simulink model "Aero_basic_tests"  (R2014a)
settings: Solver=ode1  StartTime=0.0  StopTime=inf  FixedStep=0.002  RelTol=1e-3
undefined symbols (not defined in the file or in its folder): color, HIL
libraries: quarc_library x5

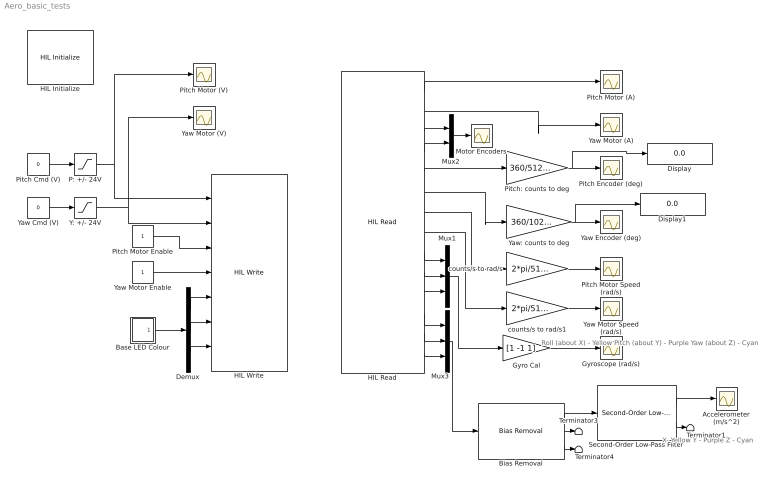
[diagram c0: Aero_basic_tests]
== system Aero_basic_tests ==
  note: Roll (about X) - Yellow Pitch (about Y) - Purple Yaw (about Z) - Cyan
  note: X- Yellow Y - Purple Z - Cyan
  Accelerometer (m/s^2) : Scope
  Base LED Colour : Subsystem
  Bias Removal : quarc_library/Discrete/Bias Removal  start_time=0  end_time=0.1  switch_id=0  sample_time=qc_get_step_size
  Demux : Demux  Outputs=3
  Display : Display
  Display1 : Display
  Gyro Cal : Gain  Gain=[1 -1 1]
  Gyroscope (rad/s) : Scope
  HIL Initialize : quarc_library/Data Acquisition/Generic/Configuration/HIL Initialize  Priority=-99  object_name=HIL-1  board_type=quanser_aero_usb  board_number=0  board_options=""  exclusive=off  active=off  hardware_clocks=[0]  clock_modes=[]  initial_clock_frequencies=[]  set_clock_params_at_start=off  set_clock_params_at_switch_in=off  set_clock_frequencies_at_start=off  set_clock_frequencies_at_switch_in=off  analog_input_channels=[0:1]  analog_input_maximums=3  analog_input_minimums=-3  set_analog_input_params_at_start=off  set_analog_input_params_at_switch_in=off  analog_output_channels=[0:1]  analog_output_maximums=24  analog_output_minimums=-24  initial_analog_outputs=[0]  final_analog_outputs=[0]  watchdog_analog_outputs=[0]  set_analog_output_params_at_start=off  set_analog_output_params_at_switch_in=off  set_analog_outputs_at_start=on  set_analog_outputs_at_switch_in=off  set_analog_outputs_at_terminate=on  set_analog_outputs_at_switch_out=off  set_analog_outputs_on_watchdog=on  digital_input_channels=[]  digital_output_channels=[0:1]  digital_output_configuration=[]  initial_digital_outputs=[1]  final_digital_outputs=[0]  watchdog_digital_outputs=[0]  set_digital_output_params_at_start=off  set_digital_output_params_at_switch_in=off  set_digital_outputs_at_start=on  set_digital_outputs_at_switch_in=off  set_digital_outputs_at_terminate=on  set_digital_outputs_at_switch_out=off  set_digital_outputs_on_watchdog=on  encoder_channels=[0:3]  quadrature=[4]  encoder_filter_frequency=[]  initial_encoder_counts=[0]  set_encoder_params_at_start=off  set_encoder_params_at_switch_in=off  set_encoder_counts_at_start=on  set_encoder_counts_at_switch_in=off  pwm_channels=[]  pwm_modes=[]  pwm_frequency=[]  pwm_configuration=[]  pwm_alignment=[]  pwm_polarity=[]  pwm_leading_deadband=[]  pwm_trailing_deadband=[]  initial_pwm_outputs=[]  final_pwm_outputs=[]  watchdog_pwm_outputs=[]  set_pwm_params_at_start=off  set_pwm_params_at_switch_in=off  set_pwm_outputs_at_start=off  set_pwm_outputs_at_switch_in=off  set_pwm_outputs_at_terminate=off  set_pwm_outputs_at_switch_out=off  set_pwm_outputs_on_watchdog=off  other_output_channels=[11000:11002]  initial_other_outputs=[0 1 0]  final_other_outputs=[1 0 0]  watchdog_other_outputs=[0 0 1]  set_other_outputs_at_start=on  set_other_outputs_at_switch_in=off  set_other_outputs_at_terminate=on  set_other_outputs_at_switch_out=off  set_other_outputs_on_watchdog=on
  HIL Read : quarc_library/Data Acquisition/Generic/Immediate I//O/HIL Read  object_name=HIL-1  analog_channels=[0:1]  encoder_channels=[0:3]  digital_channels=[]  other_channels=[14000:14001 3000:3002 4000:4002]  sample_time=qc_get_step_size  active=on  vector_output=off  data_type_mode=Inherit via back propagation  encoder_data_type=double  digital_data_type=boolean
  HIL Write : quarc_library/Data Acquisition/Generic/Immediate I//O/HIL Write  object_name=HIL-1  analog_channels=[0:1]  pwm_channels=[]  digital_channels=[0:1]  other_channels=[11000:11002]  sample_time=-1  active=off  vector_input=off
  Motor Encoders : Scope
  Mux1 : Mux  Inputs=3
  Mux2 : Mux  Inputs=2
  Mux3 : Mux  Inputs=3
  P: +/- 24V : Saturate  UpperLimit=24  LowerLimit=-24
  Pitch Cmd (V) : Constant  Value=0
  Pitch Encoder (deg) : Scope
  Pitch Motor (A) : Scope
  Pitch Motor (V) : Scope
  Pitch Motor Enable : Constant
  Pitch Motor Speed (rad/s) : Scope
  Pitch: counts to deg : Gain  Gain=360/512/4
  Second-Order Low-Pass Filter : quarc_library/Continuous/Second-Order Low-Pass Filter  params_source=Internal (dialog parameters)  input_width=2*pi*15  input_zeta=1  input_init=0
  Terminator1 : Terminator
  Terminator3 : Terminator
  Terminator4 : Terminator
  Y: +/- 24V : Saturate  UpperLimit=24  LowerLimit=-24
  Yaw Cmd (V) : Constant  Value=0
  Yaw Encoder (deg) : Scope
  Yaw Motor (A) : Scope
  Yaw Motor (V) : Scope
  Yaw Motor Enable : Constant
  Yaw Motor Speed (rad/s) : Scope
  Yaw: counts to deg : Gain  Gain=360/1024/4
  counts/s to rad/s : Gain  Gain=2*pi/512/4
  counts/s to rad/s1 : Gain  Gain=2*pi/512/4
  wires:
  Base LED Colour/1(rgb) -> Demux/1
  Demux/1 -> HIL Write/5
  Demux/2 -> HIL Write/6
  Demux/3 -> HIL Write/7
  HIL Read/4 -> Mux2/2
  HIL Read/3 -> Mux2/1
  HIL Read/5 -> Pitch: counts to deg/1
  HIL Read/6 -> Yaw: counts to deg/1
  Mux2/1 -> Motor Encoders/1
  Pitch: counts to deg/1 -> Display/1, Pitch Encoder (deg)/1
  Yaw: counts to deg/1 -> Display1/1, Yaw Encoder (deg)/1
  Y: +/- 24V/1 -> Yaw Motor (V)/1, HIL Write/2
  P: +/- 24V/1 -> HIL Write/1, Pitch Motor (V)/1
  HIL Read/1 -> Pitch Motor (A)/1
  HIL Read/2 -> Yaw Motor (A)/1
  Pitch Motor Enable/1 -> HIL Write/3
  Yaw Motor Enable/1 -> HIL Write/4
  HIL Read/11 -> Mux1/3
  HIL Read/9 -> Mux1/1
  HIL Read/10 -> Mux1/2
  Mux1/1 -> Gyro Cal/1
  HIL Read/13 -> Mux3/2
  HIL Read/12 -> Mux3/1
  HIL Read/14 -> Mux3/3
  Pitch Cmd (V)/1 -> P: +/- 24V/1
  Second-Order Low-Pass Filter/2 -> Terminator1/1
  Yaw Cmd (V)/1 -> Y: +/- 24V/1
  Bias Removal/1 -> Second-Order Low-Pass Filter/1
  Mux3/1 -> Bias Removal/1
  Bias Removal/2 -> Terminator3/1
  Bias Removal/3 -> Terminator4/1
  Gyro Cal/1 -> Gyroscope (rad/s)/1
  Second-Order Low-Pass Filter/1 -> Accelerometer (m/s^2)/1
  HIL Read/7 -> counts/s to rad/s/1
  counts/s to rad/s/1 -> Pitch Motor Speed (rad/s)/1
  HIL Read/8 -> counts/s to rad/s1/1
  counts/s to rad/s1/1 -> Yaw Motor Speed (rad/s)/1

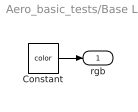
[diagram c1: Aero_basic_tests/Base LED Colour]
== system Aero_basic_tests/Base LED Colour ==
  Constant : Constant  Value=color
  rgb : Outport
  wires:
  Constant/1 -> rgb/1
